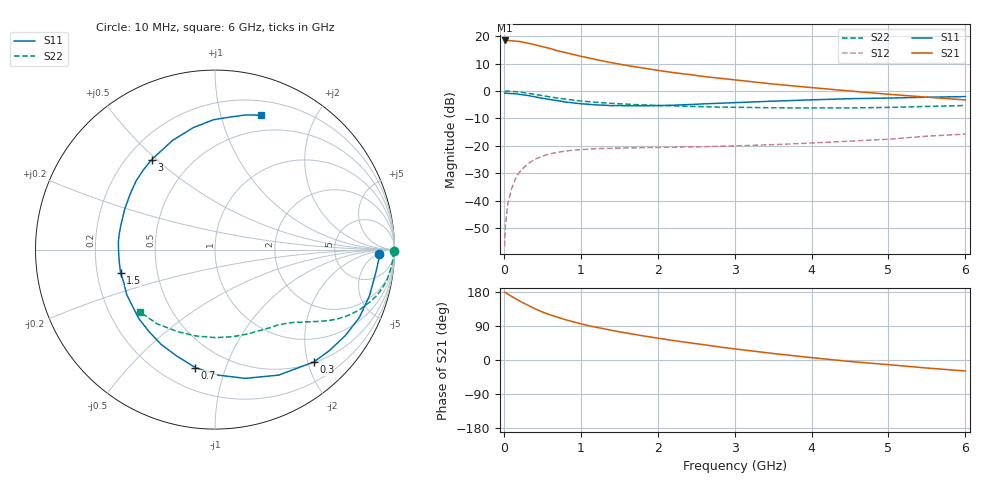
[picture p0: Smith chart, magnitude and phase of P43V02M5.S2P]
! SIEMENS Small Signal Semiconductors
! BFP182
! Si NPN RF Bipolar Junction Transistor in SOT143
! VCE = 3 V  IC = 2.5 mA
! Common Emitter S-Parameters:  March  1996
# GHz  S  MA  R  50
!  f  S11  S21  S12  S22
! GHz  MAG  ANG  MAG  ANG  MAG  ANG  MAG  ANG
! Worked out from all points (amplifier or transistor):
!   36 points, 10 MHz to 6 GHz, reference 50 ohm
!   highest |S21| = 18.4 dB at 10 MHz (marker M1)
!   |S21| within 3 dB of that: start of sweep to 609.6 MHz
!   unconditionally stable (mu >= 1): 2.036 GHz to 5.849 GHz
!   at 250 MHz: K = 0.14, MSG = 22.9 dB, |S12| = -28.1 dB
!   at 1.4 GHz: K = 0.74, MSG = 15.6 dB, |S12| = -20.9 dB
!   at 6 GHz: K = 0.98, MSG = 6.2 dB, |S12| = -15.7 dB
!   S11 on the Smith chart (normalised r, x): 10 MHz: 20, -6; 300 MHz: 0.51, -2.11; 700 MHz: 0.33, -0.79; 1.5 GHz: 0.30, -0.11; 3 GHz: 0.30, +0.48; 6 GHz: 0.34, +1.34
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0.01  0.9124 -1.7  8.308 179.0  0.0015 83.7  0.9949 -0.6
0.02  0.914 -3.5  8.301 178.2  0.0035 83.3  0.9928 -1.3
0.05  0.9049 -8.2  8.308 174.0  0.0088 86.5  0.9926 -3.3
0.1  0.8983 -16.7  8.209 168.1  0.0165 79.8  0.9831 -6.7
0.2  0.8703 -33.3  7.964 156.3  0.0329 70.8  0.9574 -12.9
0.25  0.8502 -41.5  7.728 150.8  0.0392 66.9  0.9373 -15.8
0.3  0.8335 -48.7  7.491 146.0  0.0461 63.1  0.9139 -18.4
0.4  0.7842 -63.1  6.965 135.7  0.0568 55.9  0.8696 -22.9
0.5  0.7369 -76.8  6.414 126.8  0.0651 49.1  0.8229 -26.7
0.6  0.6993 -88.7  5.937 119.4  0.0718 44.0  0.7799 -29.8
0.7  0.6662 -99.5  5.384 112.7  0.0766 39.9  0.7427 -32.2
0.9  0.6078 -119.5  4.632 100.9  0.084 33.0  0.6838 -35.9
1.1  0.573 -137.7  4.012 90.7  0.0876 28.2  0.6393 -39.0
1.3  0.5523 -153.0  3.488 82.4  0.09 24.6  0.6084 -41.6
1.5  0.5422 -165.9  3.085 74.5  0.0913 22.2  0.5849 -44.2
1.8  0.5403 175.5  2.632 64.0  0.0932 20.4  0.5592 -47.9
2.2  0.5515 155.8  2.162 51.5  0.0949 18.4  0.5364 -53.8
3  0.6133 125.1  1.595 29.3  0.1002 18.4  0.5059 -67.8
3.5  0.6528 111.2  1.338 17.2  0.1055 19.0  0.4953 -78.0
4.5  0.724 90.6  0.999 -3.9  0.1225 19.5  0.4924 -102.0
5.5  0.7699 77.1  0.772 -21.2  0.1507 18.1  0.5238 -127.8
6  0.7908 71.2  0.688 -29.0  0.1642 14.7  0.5442 -140.4
